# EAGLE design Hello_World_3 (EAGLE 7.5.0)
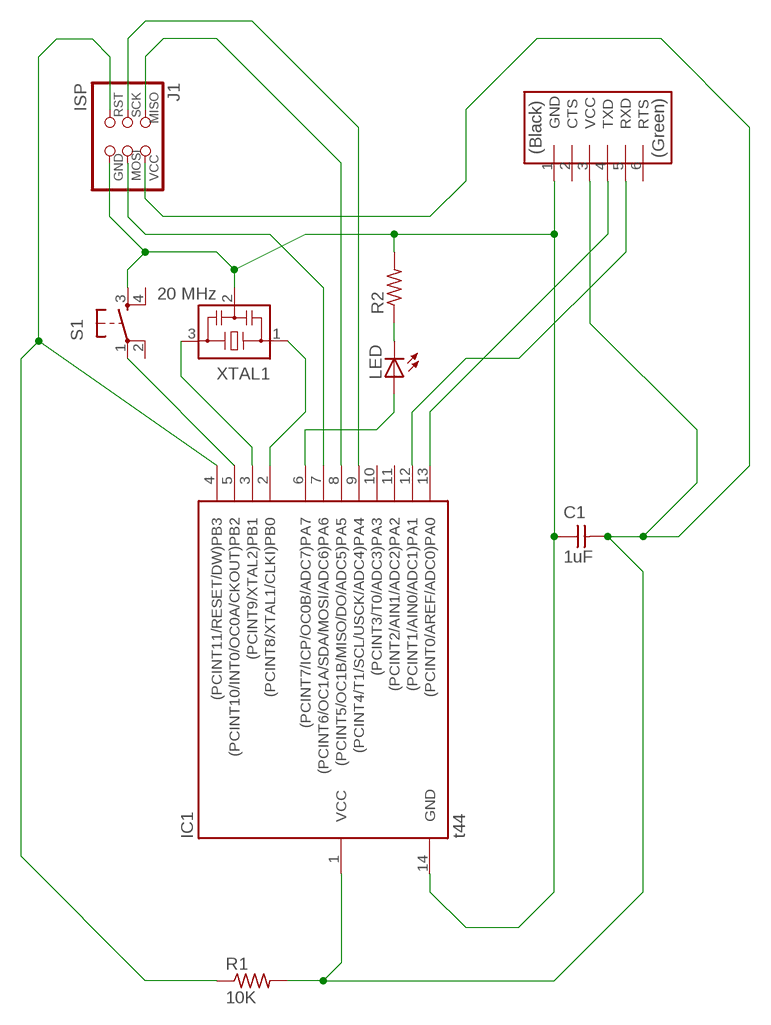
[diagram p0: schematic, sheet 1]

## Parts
C1  1uF  CAP-UNPOLARIZEDFAB  [C1206FAB]
IC1  t44  ATTINY44-SSU  [SOIC14]
J1  ISP  AVRISPSMD  [2X03SMD]
J2  FTDI  FTDI-SMD-HEADER  [1X06SMD]
LED  LEDFAB1206  [LED1206FAB]
R1  10K  RES-US1206FAB  [R1206FAB]
R2  RES-US1206FAB  [R1206FAB]
S1  6MM_SWITCH6MM_SWITCH  [6MM_SWITCH]
XTAL1  20 MHz  RESONATOR  [EFOBM]

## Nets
GND: C1.1 IC1.14(GND) J1.6(GND) J2.1(GND) R2.2 S1.3(S) XTAL1.2
N$1: IC1.5((PCINT10/INT0/OC0A/CKOUT)PB2) S1.1(P)
N$2: IC1.2((PCINT8/XTAL1/CLKI)PB0) XTAL1.1
N$3: IC1.4((PCINT11/RESET/DW)PB3) J1.5(RST) R1.1
N$4: IC1.7((PCINT6/OC1A/SDA/MOSI/ADC6)PA6) J1.4(MOSI)
N$5: IC1.8((PCINT5/OC1B/MISO/DO/ADC5)PA5) J1.1(MISO)
N$6: IC1.9((PCINT4/T1/SCL/USCK/ADC4)PA4) J1.3(SCK)
N$7: IC1.3((PCINT9/XTAL2)PB1) XTAL1.3
N$8: IC1.6((PCINT7/ICP/OC0B/ADC7)PA7) LED.1(A)
N$9: LED.2(C) R2.1
N$10: IC1.13((PCINT0/AREF/ADC0)PA0) J2.4(TXD)
N$11: IC1.12((PCINT1/AIN0/ADC1)PA1) J2.5(RXD)
VCC: C1.2 IC1.1(VCC) J1.2(VCC) J2.3(VCC) R1.2
Unconnected: IC1.10((PCINT3/T0/ADC3)PA3) IC1.11((PCINT2/AIN1/ADC2)PA2) J2.2(CTS) J2.6(RTS) S1.2(P1) S1.4(S1)

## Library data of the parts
C1 = fab:CAP-UNPOLARIZED
IC1 = fab:ATTINY44
J1 = fab:AVRISP
J2 = fab:FTDI-SMD-HEADER
LED = fab:LED: LED
R1 R2 = fab:RES-US: Resistor (US Symbol)
S1 = fab:6MM_SWITCH: OMRON SWITCH
XTAL1 = fab:RESONATOR

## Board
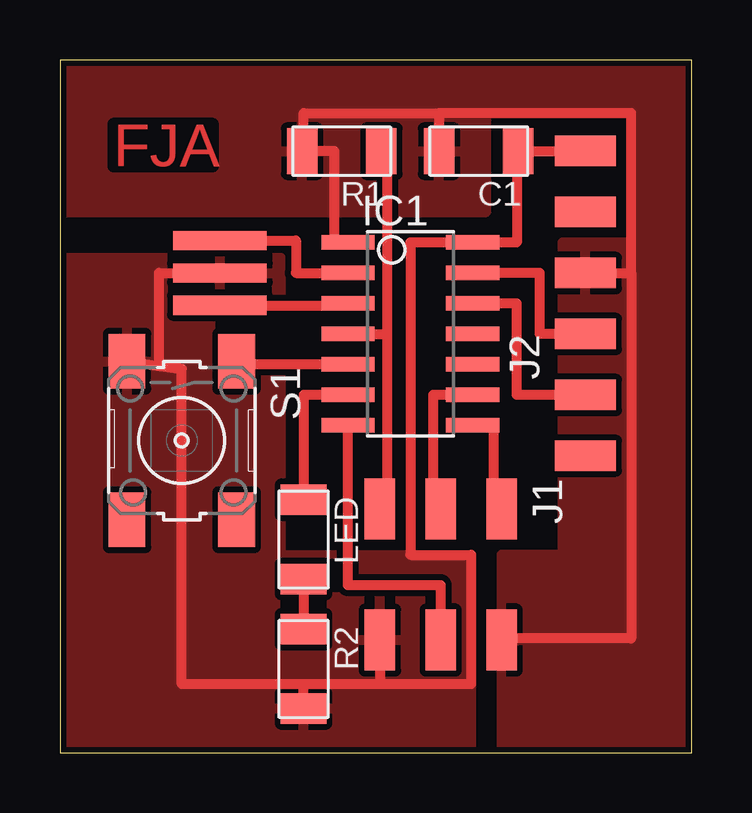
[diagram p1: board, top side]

Size 26.34 x 28.88 mm. Coordinates in mm from the lower left corner, seen from the top.
Outline: 0,0 26.34,0 26.34,28.88 0,28.88 0,0
Copper layers (1*16): Top 0.035mm / dielectric 1.5mm / Bottom 0.035mm
Design rules "MySettings *": minimum track width 6mil, minimum drill 12mil, track to track 10mil, track to pad 10mil, pad to pad 10mil, via to via 10mil, smd to smd 0mil, copper to edge 10mil, drill to drill 10mil, minimum pad ring 10mil, minimum via ring 6mil, stop-mask expansion 2mil, vias tented up to drill 100mil, thermal gap 10mil

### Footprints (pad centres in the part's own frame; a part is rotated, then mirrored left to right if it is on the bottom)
C1206FAB = smd 1.27 x 1.905: 1 -1.651,0; 2 1.651,0
SOIC14 = smd 0.61 x 2.21: 1 -3.81,-2.603; 2 -2.54,-2.603; 3 -1.27,-2.603; 4 0,-2.603; 5 1.27,-2.603; 6 2.54,-2.603; 7 3.81,-2.603; 8 3.81,2.603; 9 2.54,2.603; 10 1.27,2.603; 11 0,2.603; 12 -1.27,2.603; 13 -2.54,2.603; 14 -3.81,2.603
2X03SMD = smd 2.54 x 1.27: 1 -2.54,2.54; 2 2.92,2.54; 3 -2.54,0; 4 2.92,0; 5 -2.54,-2.54; 6 2.92,-2.54
1X06SMD = smd 2.54 x 1.27: 1 0,6.35; 2 0,3.81; 3 0,1.27; 4 0,-1.27; 5 0,-3.81; 6 0,-6.35
LED1206FAB = smd 1.27 x 1.905: 1 -1.651,0; 2 1.651,0
R1206FAB = smd 1.27 x 1.905: 1 -1.651,0; 2 1.651,0
6MM_SWITCH = smd 2.286 x 1.524: 1 -3.302,2.286; 2 3.302,2.286; 3 -3.302,-2.286; 4 3.302,-2.286
EFOBM = smd 0.8 x 3.9: 1 -1.35,0; 2 0,0; 3 1.35,0

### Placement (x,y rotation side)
C1  17.46,25.08 180 top
IC1  14.6,17.46 270 top
J1  15.87,7.62 270 top
J2  21.91,18.73 0 top
LED  10.16,8.89 270 top
R1  11.75,25.08 180 top
R2  10.16,3.49 270 top
S1  5.08,13.02 270 top
XTAL1  6.67,20 270 top

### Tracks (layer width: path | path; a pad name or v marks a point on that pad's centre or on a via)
GND
  Top 0.406: J2.1 C1.1 19.05,25.08 19.05,21.27 IC1.14 14.6,21.27 14.6,8.25 17.15,8.25 17.15,2.86 13.33,2.86 | 13.33,2.86 10.16,2.86 | 10.16,2.86 5.08,2.86 5.08,16 | XTAL1.2 4.13,20 4.13,16.19 5.08,16 | J1.6 13.33,2.86 | S1.3 5.08,16 | R2.2 10.16,2.86
  pour Top: -0.63,20.64 9.21,20.64 9.21,8.25 17.15,8.25 17.15,-0.32 -0.63,-0.32
N$1
  Top 0.406: IC1.5 7.68,16.19 S1.1
N$2
  Top 0.406: XTAL1.1 9.84,21.35 9.84,20 IC1.2
N$3
  Top 0.406: J1.5 13.65,10.16 13.65,17.46 | 13.65,17.46 13.65,23.81 13.65,24.45 13.65,25.08 R1.1 | IC1.4 13.65,17.46
N$4
  Top 0.406: J1.4 15.87,6.98 12,6.98 IC1.7
N$5
  Top 0.406: J1.1 18.1,10.16 18.1,13.65 IC1.8
N$6
  Top 0.406: IC1.9 15.56,14.92 15.56,11.11 15.87,11.11 J1.3
N$7
  Top 0.406: XTAL1.3 12,18.65 IC1.3
N$8
  Top 0.406: IC1.6 10.16,14.92 LED.1
N$9
  Top 0.406: LED.2 R2.1
N$10
  Top 0.406: J2.4 20,17.46 20,20 IC1.13
N$11
  Top 0.406: J2.5 19.05,14.92 19.05,18.73 IC1.12
VCC
  Top 0.406: R1.2 10.16,25.08 | IC1.1 11.43,21.27 11.43,25.08 10.16,25.08 | 10.16,25.08 10.16,26.67 15.81,26.67 | 15.81,26.67 C1.2 | 23.81,20 23.81,26.67 15.81,26.67 | J2.3 23.81,20 | 23.81,20 23.81,4.76 18.42,4.76 J1.2
  pour Top: 18.41,-0.32 27.3,-0.32 27.3,30.16 -0.63,30.16 -0.63,22.54 17.78,22.54 17.78,26.67 23.81,26.67 23.81,21.27 20.95,21.27 20.95,8.25 18.41,8.25

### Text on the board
Top: FJA | FJA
